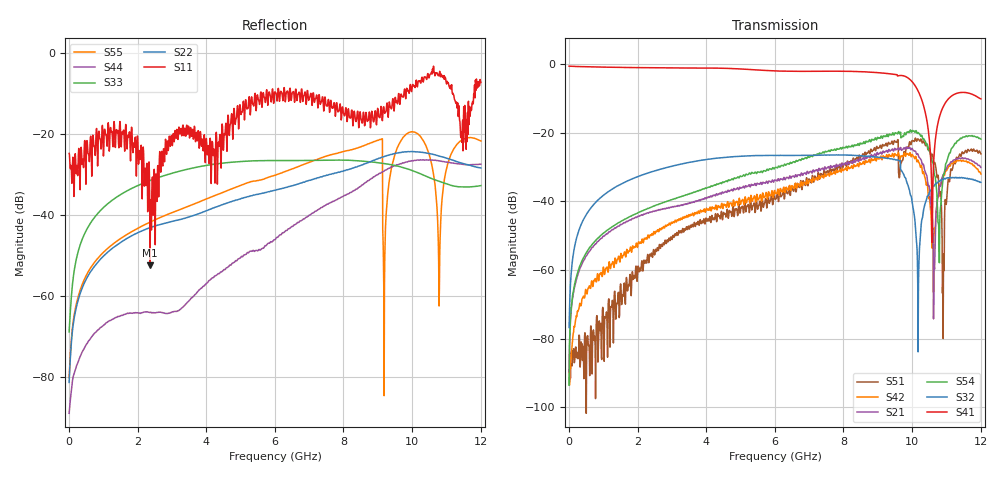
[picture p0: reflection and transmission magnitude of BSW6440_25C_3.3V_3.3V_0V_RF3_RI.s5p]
!	Test time	=	2022-08-08 18:09
!	Product	=	BSW6440
!	Temp	=	25C
!	VDD	=	3.3
!	Control_High	=	3.3
!	Control_Low	=	0
!	Logic	=	RF3
!	Porrt1	=	RFC
!	Porrt2	=	RF1
!	Porrt3	=	RF2
!	Porrt4	=	RF3
!	Porrt5	=	RF4
!	V1(LS)	=	3.3
!	V2(CTRL)	=	X
!	V3	=	X
!	V4	=	X
#	Hz	S	RI	R	50
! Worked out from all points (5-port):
!   1201 points, 5 MHz to 12.01 GHz, reference 50 ohm
!   strongest paths, dB at 5 MHz, 3.005 GHz, 6.005 GHz, 9.005 GHz, 12.01 GHz:
!     S41: -0.7, -1.2, -2.0, -2.6, -10.2
!     S32: -76.8, -29.8, -26.7, -27.2, -34.5
!     S54: -93.6, -39.5, -30.2, -21.4, -21.9
!     S21: -89.6, -41.6, -33.9, -26.3, -30.1
!     S42: -89.1, -46.4, -37.2, -27.5, -32.1
!     S51: -91.5, -51.2, -39.5, -24.7, -26.2
!   lowest |S11| = -52.5 dB at 2.365 GHz (marker M1), VSWR 1.00, Z = 49.8 + j0.064 ohm
!   |S11| at or under -10 dB: start of sweep to 5.584 GHz; 7.125 GHz to 9.763 GHz (2.638 GHz wide, 31.2 % of centre); 11.19 GHz to 11.81 GHz (623.2 MHz wide, 5.42 % of centre)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
